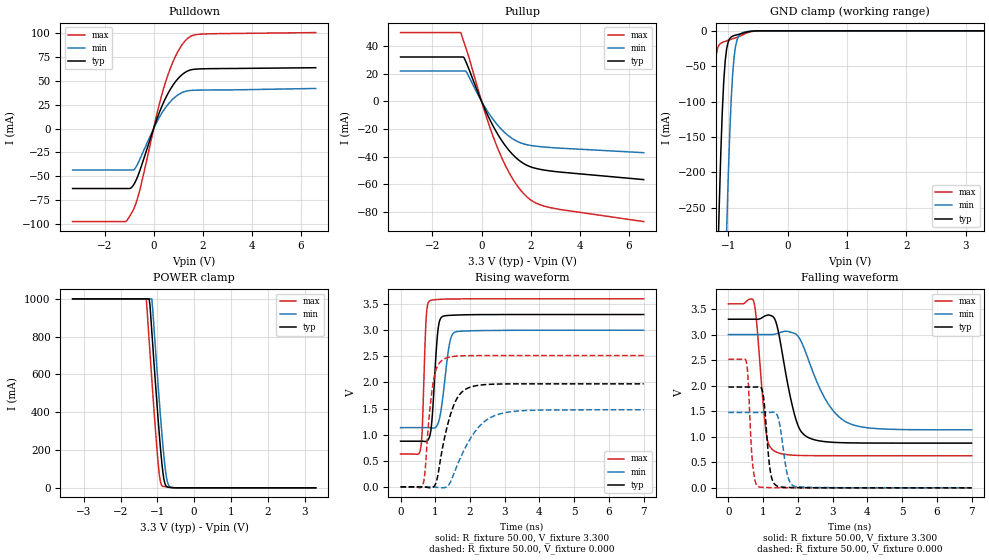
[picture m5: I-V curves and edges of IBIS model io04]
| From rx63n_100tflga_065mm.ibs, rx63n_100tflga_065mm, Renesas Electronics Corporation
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[Model]   io04
Model_type   I/O
Polarity   Non-Inverting
Enable   Active-High
Vinl  =   0.660V
Vinh  =   2.640V
Vmeas =   1.650V
Cref  =   30.00pF
| variable   typ   min   max
C_comp   4.420pF   4.420pF   4.420pF
| variable   typ   min   max
[Temperature Range]   45.000   105.000   -40.000
| variable   typ   min   max
[Voltage Range]   3.300V   3.000V   3.600V
| variable   typ   min   max
[Pullup Reference]   3.300V   3.000V   3.600V
| variable   typ   min   max
[Pulldown Reference]   0.000V   0.000V   0.000V
| variable   typ   min   max
[POWER Clamp Reference] 3.300V   3.000V   3.600V
| variable   typ   min   max
[GND Clamp Reference]   0.000V   0.000V   0.000V
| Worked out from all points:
|   slope of the pulldown table from 0 to 0.495 V, typ, clamps not added: 15.4 ohm
|   slope of the pullup table from 0 to 0.495 V, typ, clamps not added: 26.5 ohm
|   GND clamp passes 1 mA (typ) near -0.64 V on its own axis
|   POWER clamp passes 1 mA (typ) near -0.59 V on its own axis
|   rising waveform, R_fixture 50.00, V_fixture 3.300: 20-80 % time 137ps typ, 205ps min, 88.9ps max; typ from 0.875 V to 3.3 V
|   rising waveform, R_fixture 50.00, V_fixture 0.000: 20-80 % time 423ps typ, 741ps min, 213ps max; typ from 0 V to 1.97 V
|   falling waveform, R_fixture 50.00, V_fixture 3.300: 20-80 % time 429ps typ, 779ps min, 219ps max; typ from 3.3 V to 0.875 V
|   falling waveform, R_fixture 50.00, V_fixture 0.000: 20-80 % time 149ps typ, 194ps min, 116ps max; typ from 1.97 V to 0 V
[Pulldown]
| io04_strong Pulldown rx631_rx63n
| Thu Mar 22 17:15:49 2012
| voltage   I(typ)   I(min)   I(max)
-3.3V     -62.62mA   -43.25mA   -97.14mA
-1.15V    -62.62mA   -43.25mA   -97.14mA
-1.025V   -62.62mA   -43.25mA   -93.52mA
-800mV    -58.13mA   -42.94mA   -83.32mA
-600mV    -46.6mA    -34.2mA    -67.76mA
175mV     12.96mA    9.062mA    19.78mA
550mV     35.03mA    24.16mA    53.68mA
950mV     50.91mA    34.42mA    78.65mA
1.4V      60.32mA    39.47mA    94.53mA
1.7V      62.04mA    40.07mA    97.97mA
2.1V      62.47mA    40.25mA    98.84mA
6.6V      63.56mA    41.89mA    100.3mA
[Pullup]
| io04_strong Pullup rx631_rx63n
| Thu Mar 22 17:15:49 2012
| voltage   I(typ)   I(min)   I(max)
-3.3V     32.04mA    21.95mA    49.68mA
-850mV    32.04mA    21.95mA    49.68mA
-725mV    31.77mA    21.95mA    43.08mA
-625mV    28.06mA    21.43mA    37.88mA
150mV     -6.165mA   -4.558mA   -8.71mA
675mV     -24.25mA   -17.59mA   -34.7mA
1V        -32.82mA   -23.46mA   -47.4mA
1.3V      -39mA      -27.43mA   -56.91mA
1.925V    -46.81mA   -31.61mA   -70.21mA
2.3V      -48.81mA   -32.55mA   -74.14mA
2.9V      -50.5mA    -33.47mA   -77.15mA
6.6V      -56.53mA   -37.08mA   -86.83mA
[GND Clamp]
| io04_strong GNDClamp rx631_rx63n
| Thu Mar 22 17:15:49 2012
| voltage   I(typ)   I(min)   I(max)
-3.3V     -1A        -1A        -1A
-1.325V   -916.4mA   -1A        -321.6mA
-1.225V   -508.3mA   -1A        -56.05mA
-1.175V   -327.1mA   -831.8mA   -23.6mA
-1.15V    -246.5mA   -730.6mA   -19.51mA
-1.075V   -71.99mA   -445.9mA   -15.62mA
-1.025V   -24.89mA   -280.5mA   -14.09mA
-975mV    -11.12mA   -147.9mA   -12.65mA
-925mV    -7.484mA   -61.53mA   -11.26mA
-850mV    -5.559mA   -12.59mA   -9.146mA
-675mV    -1.555mA   -930uA     -2.738mA
3.3V      0A         0A         0A
[POWER Clamp]
| io04_strong PWRClamp rx631_rx63n
| Thu Mar 22 17:15:49 2012
| voltage   I(typ)   I(min)   I(max)
-3.3V     1A         1A         1A
-1.3V     1A         1A         1A
-1.225V   1A         1A         787.8mA
-1.2V     968.8mA    1A         716.2mA
-1.15V    827mA      1A         574.7mA
-975mV    353.5mA    532.6mA    124.6mA
-925mV    232.2mA    403.9mA    41.33mA
-875mV    126.2mA    282.6mA    11.35mA
-825mV    48.99mA    173.5mA    7.014mA
-750mV    7.221mA    53mA       4.912mA
-625mV    1.442mA    2.321mA    1.9mA
3.3V      0A         0A         0A
[Ramp]
dV/dt_r   1.184/423.57p  0.886/740.07p  1.509/212.85p
dV/dt_f   1.455/428.81p  1.119/778.62p  1.783/218.73p
R_load = 50.00ohm
[Rising Waveform]
| io04_strong Rising-High rx631_rx63n
| Thu Mar 22 17:15:49 2012
R_fixture = 50.00
V_fixture = 3.300
V_fixture_min = 3.000
V_fixture_max = 3.600
C_fixture = 0.00pF
| Time   V(typ)   V(min)   V(max)
0s        875mV      1.135V     628mV
575ps     876mV      1.135V     720mV
625ps     875mV      1.135V     1.101V
740ps     871mV      1.136V     3.247V
840ps     969mV      1.134V     3.562V
1.075ns   2.982V     1.207V     3.588V
1.205ns   3.261V     1.649V     3.593V
1.4ns     3.283V     2.704V     3.597V
1.57ns    3.289V     2.964V     3.599V
7ns       3.3V       3V         3.6V
[Rising Waveform]
| io04_strong Rising-Low rx631_rx63n
| Thu Mar 22 17:15:49 2012
R_fixture = 50.00
V_fixture = 0.000
C_fixture = 0.00pF
| Time   V(typ)   V(min)   V(max)
0s        0V         0V         0V
655ps     0V         0V         70mV
835ps     -17mV      0V         1.423V
945ps     1mV        -2mV       2.018V
1.06ns    173mV      -9mV       2.308V
1.245ns   869mV      -16mV      2.444V
1.705ns   1.772V     526mV      2.508V
2.195ns   1.94V      1.102V     2.514V
2.685ns   1.967V     1.358V     2.515V
7ns       1.973V     1.476V     2.515V
[Falling Waveform]
| io04_strong Falling-High rx631_rx63n
| Thu Mar 22 17:15:49 2012
R_fixture = 50.00
V_fixture = 3.300
V_fixture_min = 3.000
V_fixture_max = 3.600
C_fixture = 0.00pF
| Time   V(typ)   V(min)   V(max)
0s        3.3V       3V         3.6V
730ps     3.3V       3V         3.645V
810ps     3.299V     3V         3.25V
1.09ns    3.374V     3V         1.055V
1.325ns   3.313V     3.004V     720mV
1.91ns    1.416V     3.019V     637mV
2.245ns   1.005V     2.613V     631mV
2.85ns    899mV      1.667V     629mV
3.43ns    881mV      1.275V     628mV
7ns       875mV      1.135V     628mV
[Falling Waveform]
| io04_strong Falling-Low rx631_rx63n
| Thu Mar 22 17:15:49 2012
R_fixture = 50.00
V_fixture = 0.000
C_fixture = 0.00pF
| Time   V(typ)   V(min)   V(max)
0s        1.973V     1.476V     2.515V
515ps     1.973V     1.476V     2.467V
695ps     1.973V     1.476V     474mV
845ps     1.975V     1.476V     28mV
1ns       1.82V      1.476V     10mV
1.225ns   253mV      1.478V     4mV
1.415ns   31mV       1.405V     2mV
1.69ns    9mV        278mV      1mV
1.9ns     5mV        31mV       0V
7ns       0V         0V         0V
